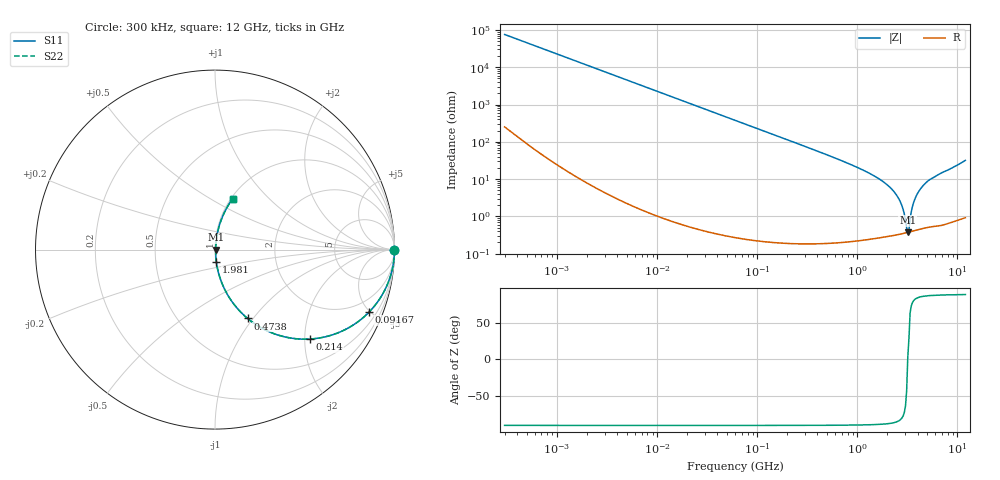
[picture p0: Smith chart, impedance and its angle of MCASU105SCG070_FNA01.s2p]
! MCASU105SCG070_FNA01  S-PARAMETER MODEL  ( Standard Model )
! Model Generated by TAIYO YUDEN Corporation (http://www.ty-top.com)
! Version 1.0
! TAIYO YUDEN Control No. 230609
! Copyright(c) 2023 TAIYO YUDEN CO.,LTD. All Rights Reserved.
! Product Description (link to TY-COMPAS)
! https://ds.yuden.co.jp/TYCOMPAS/or/detail?pn=MCASU105SCG070CFNA01&u=M
! Products Name : Multilayer Ceramic Capacitors
! Characteristics :
!  Capacitance : 7 [pF] , Rated Voltage : 50 [V] , TCC : CG / C0G
!  Case Size : 1.0 x 0.5 / 0.039 x 0.02 [mm/inch] , Thickness : 0.5 / 0.02 [mm/inch]
!  (Conditions: Temperature = 25 [degC] , DC Bias Voltage = 0 [V])
! External Node Assignments :
!  1  o---| |---o  2
! GND o---------o GND
! Frequency Range : 0.3MHz  -  12000MHz  [ 401 STEP ]
# MHZ S RI R 50
! Freq[MHz].  S11 Real  S11 Imag  S21 Real  S21 Imag  S12 Real  S12 Imag  S22 Real  S22 Imag
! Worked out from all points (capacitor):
!   401 points, 300 kHz to 12 GHz, reference 50 ohm
!   read as one part in series: C = 7 pF near 316.3 kHz
!   lowest |Z| = 370 mohm at 3.191 GHz (marker M1)
!   series resonance near 3.186 GHz, so ESL is about 360 pH
!   S11 on the Smith chart (normalised r, x): 300 kHz: open; 91.67 MHz: 1.00, -4.96; 214 MHz: 1.00, -2.12; 473.8 MHz: 1.00, -0.94; 1.981 GHz: 1.01, -0.14; 12 GHz: 1.02, +0.63
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0.3  1 -0.00132  6.1e-06 0.00132  6.1e-06 0.00132  1 -0.00132
1.769972  0.9999 -0.00778  6.63e-05 0.00778  6.63e-05 0.00778  0.9999 -0.00778
10.44266  0.9979 -0.0458  0.00213 0.0458  0.00213 0.0458  0.9979 -0.0458
60  0.9347 -0.2467  0.0653 0.2467  0.0653 0.2467  0.9347 -0.2467
91.67136  0.8597 -0.3468  0.1403 0.3468  0.1403 0.3468  0.8597 -0.3468
213.9924  0.528 -0.4983  0.472 0.4983  0.472 0.4983  0.528 -0.4983
353.9943  0.2875 -0.4512  0.7125 0.4512  0.7125 0.4512  0.2875 -0.4512
473.7541  0.1814 -0.3834  0.8186 0.3834  0.8186 0.3834  0.1814 -0.3834
1135.593  0.0317 -0.1688  0.9683 0.1688  0.9683 0.1688  0.0317 -0.1688
1980.756  0.00771 -0.0696  0.9923 0.0696  0.9923 0.0696  0.00771 -0.0696
2088.533  0.0067 -0.0614  0.9933 0.0614  0.9933 0.0614  0.0067 -0.0614
2650.866  0.00396 -0.026  0.996 0.026  0.996 0.026  0.00396 -0.026
2870.14  0.00365 -0.0146  0.9963 0.0146  0.9963 0.0146  0.00365 -0.0146
3107.553  0.00363 -0.00333  0.9964 0.00333  0.9964 0.00333  0.00363 -0.00333
3190.978  0.00368 0.000204  0.9963 -0.000204  0.9963 -0.000204  0.00368 0.000204
3364.605  0.00387 0.00755  0.9961 -0.00755  0.9961 -0.00755  0.00387 0.00755
3547.679  0.00426 0.0174  0.9957 -0.0174  0.9957 -0.0174  0.00426 0.0174
3740.715  0.00488 0.0276  0.9951 -0.0276  0.9951 -0.0276  0.00488 0.0276
4050.141  0.00623 0.0432  0.9938 -0.0432  0.9938 -0.0432  0.00623 0.0432
4623.766  0.00956 0.069  0.9904 -0.069  0.9904 -0.069  0.00956 0.069
6524.734  0.0228 0.1302  0.9772 -0.1302  0.9772 -0.1302  0.0228 0.1302
12000  0.0983 0.2837  0.9017 -0.2837  0.9017 -0.2837  0.0983 0.2837
